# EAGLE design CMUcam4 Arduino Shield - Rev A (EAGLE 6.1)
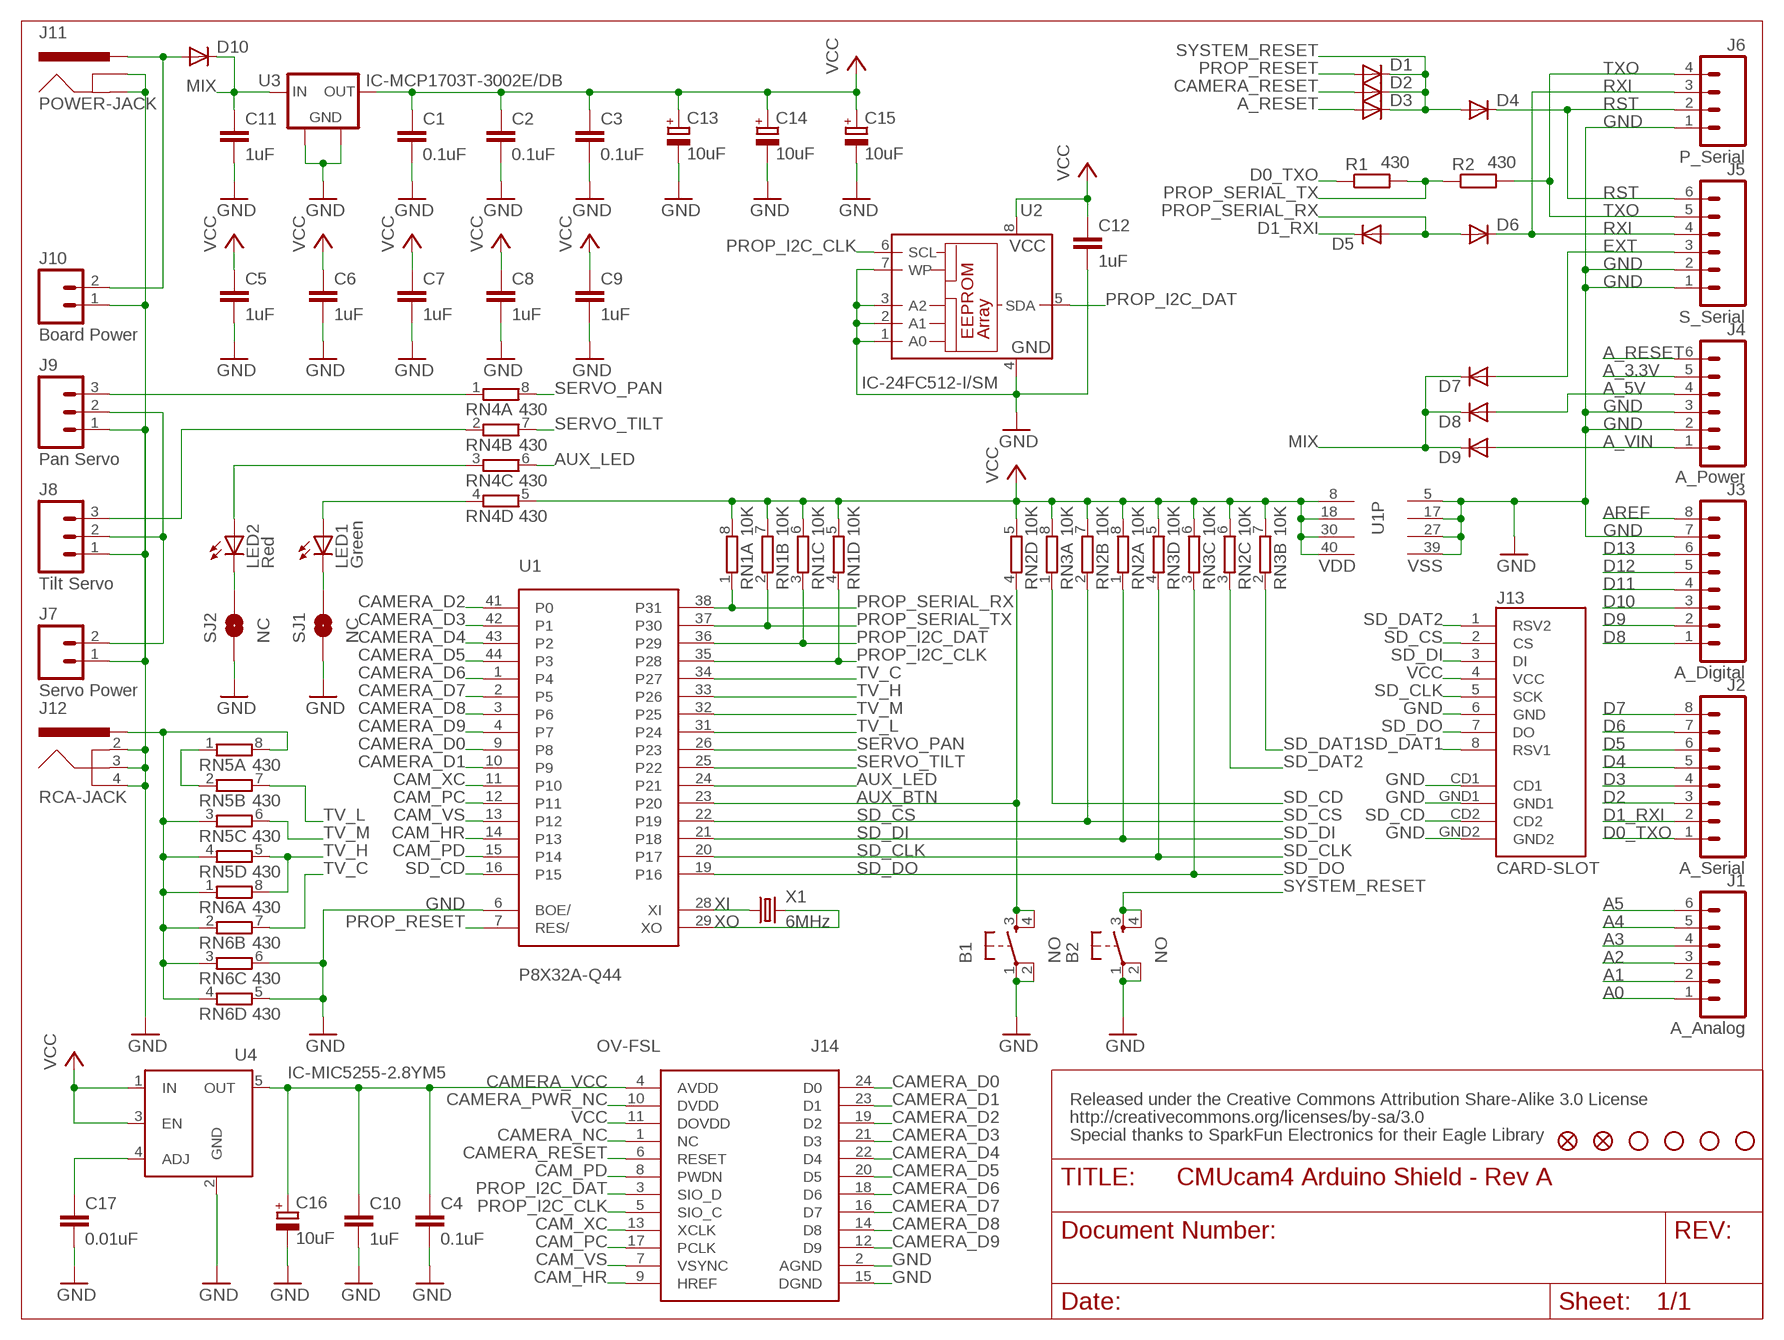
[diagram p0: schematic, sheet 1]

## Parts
B1  NO  PUSH-BUTTON  [PUSH-BUTTON]
B2  NO  PUSH-BUTTON  [PUSH-BUTTON]
C1  0.1uF  C-EUC0603K  [C0603K]
C2  0.1uF  C-EUC0603K  [C0603K]
C3  0.1uF  C-EUC0603K  [C0603K]
C4  0.1uF  C-EUC0603K  [C0603K]
C5  1uF  C-EUC0603K  [C0603K]
C6  1uF  C-EUC0603K  [C0603K]
C7  1uF  C-EUC0603K  [C0603K]
C8  1uF  C-EUC0603K  [C0603K]
C9  1uF  C-EUC0603K  [C0603K]
C10  1uF  C-EUC0603K  [C0603K]
C11  1uF  C-EUC0603K  [C0603K]
C12  1uF  C-EUC0603K  [C0603K]
C13  10uF  CPOL-EUA/3216-18R  [A/3216-18R]
C14  10uF  CPOL-EUA/3216-18R  [A/3216-18R]
C15  10uF  CPOL-EUA/3216-18R  [A/3216-18R]
C16  10uF  CPOL-EUA/3216-18R  [A/3216-18R]
C17  0.01uF  C-EUC0603K  [C0603K]
D1  DIODE-SOD523  [SOD523]
D2  DIODE-SOD523  [SOD523]
D3  DIODE-SOD523  [SOD523]
D4  DIODE-SOD523  [SOD523]
D5  DIODE-SOD523  [SOD523]
D6  DIODE-SOD523  [SOD523]
D7  DIODE-SOD323-R  [SOD323]
D8  DIODE-SOD323-R  [SOD323]
D9  DIODE-SOD323-R  [SOD323]
D10  DIODE-SOD323-R  [SOD323]
FID1  FIDUCIAL1X2  [FIDUCIAL-1X2]
FID2  FIDUCIAL1X2  [FIDUCIAL-1X2]
J1  A_Analog  M06SIP  [1X06]
J2  A_Serial  M081X08  [1X08]
J3  A_Digital  M081X08  [1X08]
J4  A_Power  M06SIP  [1X06]
J5  S_Serial  M06SIP  [1X06]
J6  P_Serial  M04PTH  [1X04]
J7  Servo Power  M02PTH  [1X02]
J8  Tilt Servo  M03PTH  [1X03]
J9  Pan Servo  M03PTH  [1X03]
J10  Board Power  M02PTH  [1X02]
J11  POWER-JACK  [POWER-JACK]
J12  RCA-JACK  [RCA-JACK]
J13  CARD-SLOT  [CARD-SLOT]
J14  OV-FSL  [OV-FSL]
LED1  Green  LEDCHIP-LED0603  [CHIP-LED0603]
LED2  Red  LEDCHIP-LED0603  [CHIP-LED0603]
R1  430  R-EU_R0603  [R0603]
R2  430  R-EU_R0603  [R0603]
RN1  10K  4R-N0603-ARV  [0603-ARV]
RN2  10K  4R-N0603-ARV  [0603-ARV]
RN3  10K  4R-N0603-ARV  [0603-ARV]
RN4  430  4R-N0603-ARV  [0603-ARV]
RN5  430  4R-N0603-ARV  [0603-ARV]
RN6  430  4R-N0603-ARV  [0603-ARV]
SJ1  NC  SOLDERJUMPERTRACE  [SJ_2S-TRACE]
SJ2  NC  SOLDERJUMPERTRACE  [SJ_2S-TRACE]
STD1  STAND-OFF  [STAND-OFF]
STD2  STAND-OFF  [STAND-OFF]
STD3  STAND-OFF  [STAND-OFF]
STD4  STAND-OFF  [STAND-OFF]
U1  P8X32A-Q44  [P8X32A-Q44]
U2  IC-24FC512-I/SM  [IC-SO-08M]
U3  IC-MCP1703T-3002E/DB  [IC-SOT-223]
U4  IC-MIC5255-2.8YM5  [IC-SOT-23-5]
X1  6MHz  CRYSTALHC49UP  [HC49UP]

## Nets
A0: J1.1
A1: J1.2
A2: J1.3
A3: J1.4
A4: J1.5
A5: J1.6
A_3.3V: J4.5
A_5V [vcc]: D8.A J4.4
A_RESET: D3.A J4.6
A_VIN: D9.A J4.1
AREF: J3.8
AUX_BTN: B1.3 B1.4 RN2.4 U1.23(P20)
AUX_LED: RN4.6 U1.24(P21)
BYP: C17.1 U4.4(ADJ)
CAM_HR: J14.9(HREF) U1.14(P13)
CAM_PC: J14.17(PCLK) U1.12(P11)
CAM_PD: J14.8(PWDN) U1.15(P14)
CAM_VS: J14.7(VSYNC) U1.13(P12)
CAM_XC: J14.13(XCLK) U1.11(P10)
CAMERA_D0: J14.24(D0) U1.9(P8)
CAMERA_D1: J14.23(D1) U1.10(P9)
CAMERA_D2: J14.19(D2) U1.41(P0)
CAMERA_D3: J14.21(D3) U1.42(P1)
CAMERA_D4: J14.22(D4) U1.43(P2)
CAMERA_D5: J14.20(D5) U1.44(P3)
CAMERA_D6: J14.18(D6) U1.1(P4)
CAMERA_D7: J14.16(D7) U1.2(P5)
CAMERA_D8: J14.14(D8) U1.3(P6)
CAMERA_D9: J14.12(D9) U1.4(P7)
CAMERA_NC: J14.1(NC)
CAMERA_PWR_NC: J14.10(DVDD)
CAMERA_RESET: D2.A J14.6(RESET)
CAMERA_VCC: C4.1 C10.1 C16.+ J14.4(AVDD) U4.5(OUT)
D0_TXO: J2.1 R1.1
D1_RXI: D5.C J2.2
D2: J2.3
D3: J2.4
D4: J2.5
D5: J2.6
D6: J2.7
D7: J2.8
D8: J3.1
D9: J3.2
D10: J3.3
D11: J3.4
D12: J3.5
D13: J3.6
EXT: D7.A J5.3
GND [vcc]: B1.1 B1.2 B2.1 B2.2 C1.2 C2.2 C3.2 C4.2 C5.2 C6.2 C7.2 C8.2 C9.2 C10.2 C11.2 C12.2 C13.- C14.- C15.- C16.- C17.2 J3.7 J4.2 J4.3 J5.1 J5.2 J6.1 J7.1 J8.1 J9.1 J10.1 J11.GND J11.GNDBREAK J12.2 J12.3 J12.4 J13.6(GND) J13.CD1 J13.GND1 J13.GND2 J14.2(AGND) J14.15(DGND) RN6.5 RN6.6 SJ1.1 SJ2.1 U1.5(VSS) U1.6(BOE/) U1.17(VSS) U1.27(VSS) U1.39(VSS) U2.1(A0) U2.2(A1) U2.3(A2) U2.4(GND) U2.7(WP) U3.2(GND) U3.4(FGND) U4.2(GND)
GREEN_BRIDGE: LED1.C SJ1.2
GREEN_CTRL: LED1.A RN4.4
MIX: C11.1 D7.C D8.C D9.C D10.C U3.1(IN)
PROP_I2C_CLK: J14.5(SIO_C) RN1.4 U1.35(P28) U2.6(SCL)
PROP_I2C_DAT: J14.3(SIO_D) RN1.3 U1.36(P29) U2.5(SDA)
PROP_RESET: D1.A U1.7(RES/)
PROP_SERIAL_RX: D5.A D6.A RN1.1 U1.38(P31)
PROP_SERIAL_TX: R1.2 R2.1 RN1.2 U1.37(P30)
RED_BRIDGE: LED2.C SJ2.2
RED_CTRL: LED2.A RN4.3
RST: D4.C J5.6 J6.2
RXI: D6.C J5.4 J6.3
SD_CD: J13.CD2 RN3.1 U1.16(P15)
SD_CLK: J13.5(SCK) RN3.4 U1.20(P17)
SD_CS: J13.2(CS) RN2.2 U1.22(P19)
SD_DAT1: J13.8(RSV1) RN3.2
SD_DAT2: J13.1(RSV2) RN2.3
SD_DI: J13.3(DI) RN2.1 U1.21(P18)
SD_DO: J13.7(DO) RN3.3 U1.19(P16)
SERVO_PAN: RN4.8 U1.26(P23)
SERVO_PAN_IO: J9.3 RN4.1
SERVO_PWR: J7.2 J8.2 J9.2
SERVO_TILT: RN4.7 U1.25(P22)
SERVO_TILT_IO: J8.3 RN4.2
SYSTEM_RESET: B2.3 B2.4 D1.C D2.C D3.C D4.A
SYSTEM_VIN: D10.A J10.2 J11.PWR
TV: J12.1 RN5.3 RN5.4 RN5.8 RN6.1 RN6.2 RN6.3 RN6.4
TV_C: RN6.7 U1.34(P27)
TV_H: RN5.5 RN6.8 U1.33(P26)
TV_L: RN5.7 U1.31(P24)
TV_M: RN5.6 U1.32(P25)
TV_R: RN5.1 RN5.2
TXO: J5.5 J6.4 R2.2
VCC: C1.1 C2.1 C3.1 C5.1 C6.1 C7.1 C8.1 C9.1 C12.1 C13.+ C14.+ C15.+ J13.4(VCC) J14.11(DOVDD) RN1.5 RN1.6 RN1.7 RN1.8 RN2.5 RN2.6 RN2.7 RN2.8 RN3.5 RN3.6 RN3.7 RN3.8 RN4.5 U1.8(VDD) U1.18(VDD) U1.30(VDD) U1.40(VDD) U2.8(VCC) U3.3(OUT) U4.1(IN) U4.3(EN)
XI: U1.28(XI) X1.1
XO: U1.29(XO) X1.2

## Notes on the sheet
- Released under the Creative Commons Attribution Share-Alike 3.0 License
- http://creativecommons.org/licenses/by-sa/3.0
- Special thanks to SparkFun Electronics for their Eagle Library

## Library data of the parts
B1 B2 = custom-jacks:PUSH-BUTTON
C1-C12 C17 = resistor:C-EU: CAPACITOR, European symbol
C13-C16 = resistor:CPOL-EU: POLARIZED CAPACITOR, European symbol
D1-D10 = diode:DIODE-: DIODE
FID1 FID2 = SparkFun:FIDUCIAL: Fiducial Alignment Points
J1 J4 J5 = SparkFun:M06: Header 6 Standard 6-pin 0.1" header. Use with straight break away headers (SKU : PRT-00116), right angle break away headers (PRT-00553), swiss pins (PRT-00743), machine pins (PRT-00117), and female headers (PRT-00115). Molex polarized connector foot print use with SKU : PRT-08094 with associated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
J2 J3 = SparkFun:M08: Header 8 Standard 8-pin 0.1" header. Use with straight break away headers (SKU : PRT-00116), right angle break away headers (PRT-00553), swiss pins (PRT-00743), machine pins (PRT-00117), and female headers (PRT-00115).
J6 = SparkFun:M04: Header 4 Standard 4-pin 0.1" header. Use with straight break away headers (SKU : PRT-00116), right angle break away headers (PRT-00553), swiss pins (PRT-00743), machine pins (PRT-00117), and female headers (PRT-00115). Molex polarized connector foot print use with SKU : PRT-08231 with associated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
J7 J10 = SparkFun:M02: Header 2
J8 J9 = SparkFun:M03: Header 3 Standard 3-pin 0.1" header. Use with straight break away headers (SKU : PRT-00116), right angle break away headers (PRT-00553), swiss pins (PRT-00743), machine pins (PRT-00117), and female headers (PRT-00115). Molex polarized connector foot print use with SKU : PRT-08232 with associated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
J11 = custom-jacks:POWER-JACK
J12 = custom-jacks:RCA-JACK
J13 = custom-jacks:CARD-SLOT
J14 = ovt-breakout:OV-FSL
LED1 LED2 = led:LED: LED
R1 R2 = resistor:R-EU_: RESISTOR, European symbol
RN1-RN6 = resistor-dil:4R-N: Array Chip Resistor Source: RS Component / Phycomp; OC_FARNELL: unknown; OC_NEWARK: unknown
SJ1 SJ2 = SparkFun:SOLDERJUMPER: Solder Jumper
STD1-STD4 = SparkFun:STAND-OFF: Stand Off
U1 = parallax-propeller:P8X32A-Q44
U2 = custom-jacks:IC-24FC512-I/SM
U3 = custom-jacks:IC-MCP1703T-3002E/DB
U4 = custom-jacks:IC-MIC5255-2.8YM5
X1 = crystal:CRYSTAL: CRYSTAL; OC_FARNELL: unknown; OC_NEWARK: unknown

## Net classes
0 default: width 0.203 mm
1 vcc: width 0.254 mm

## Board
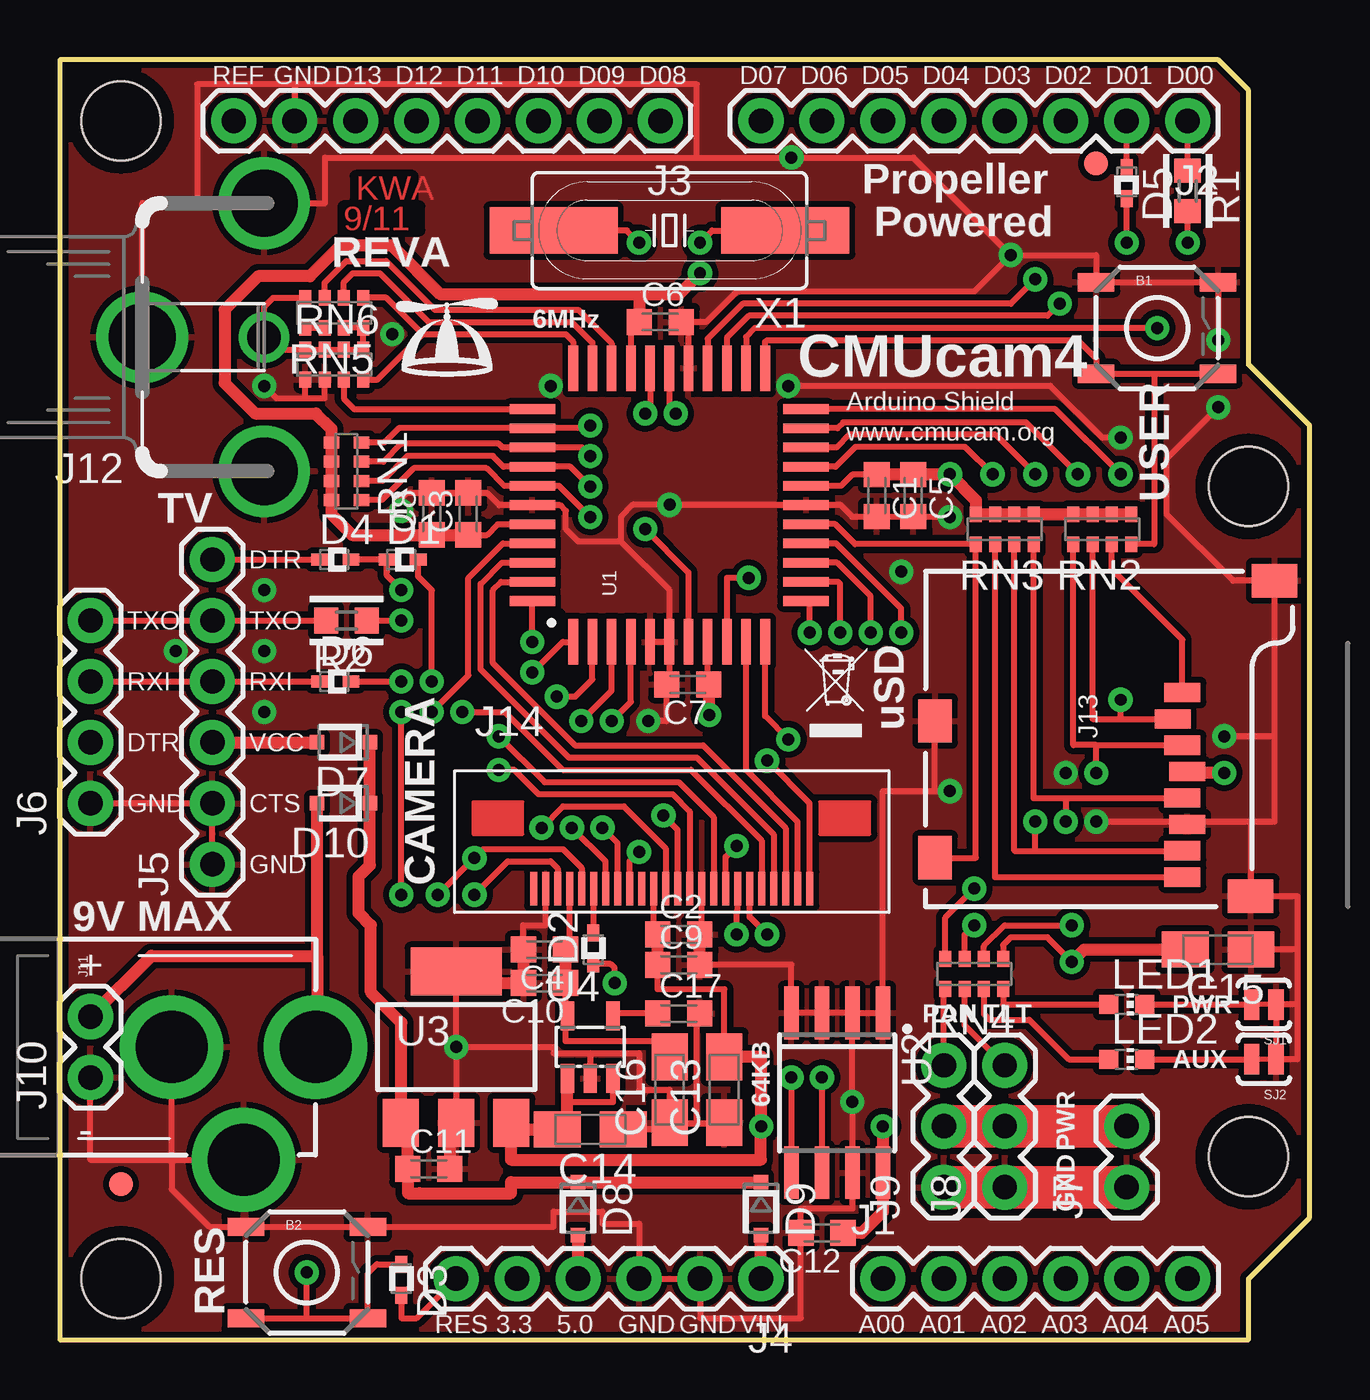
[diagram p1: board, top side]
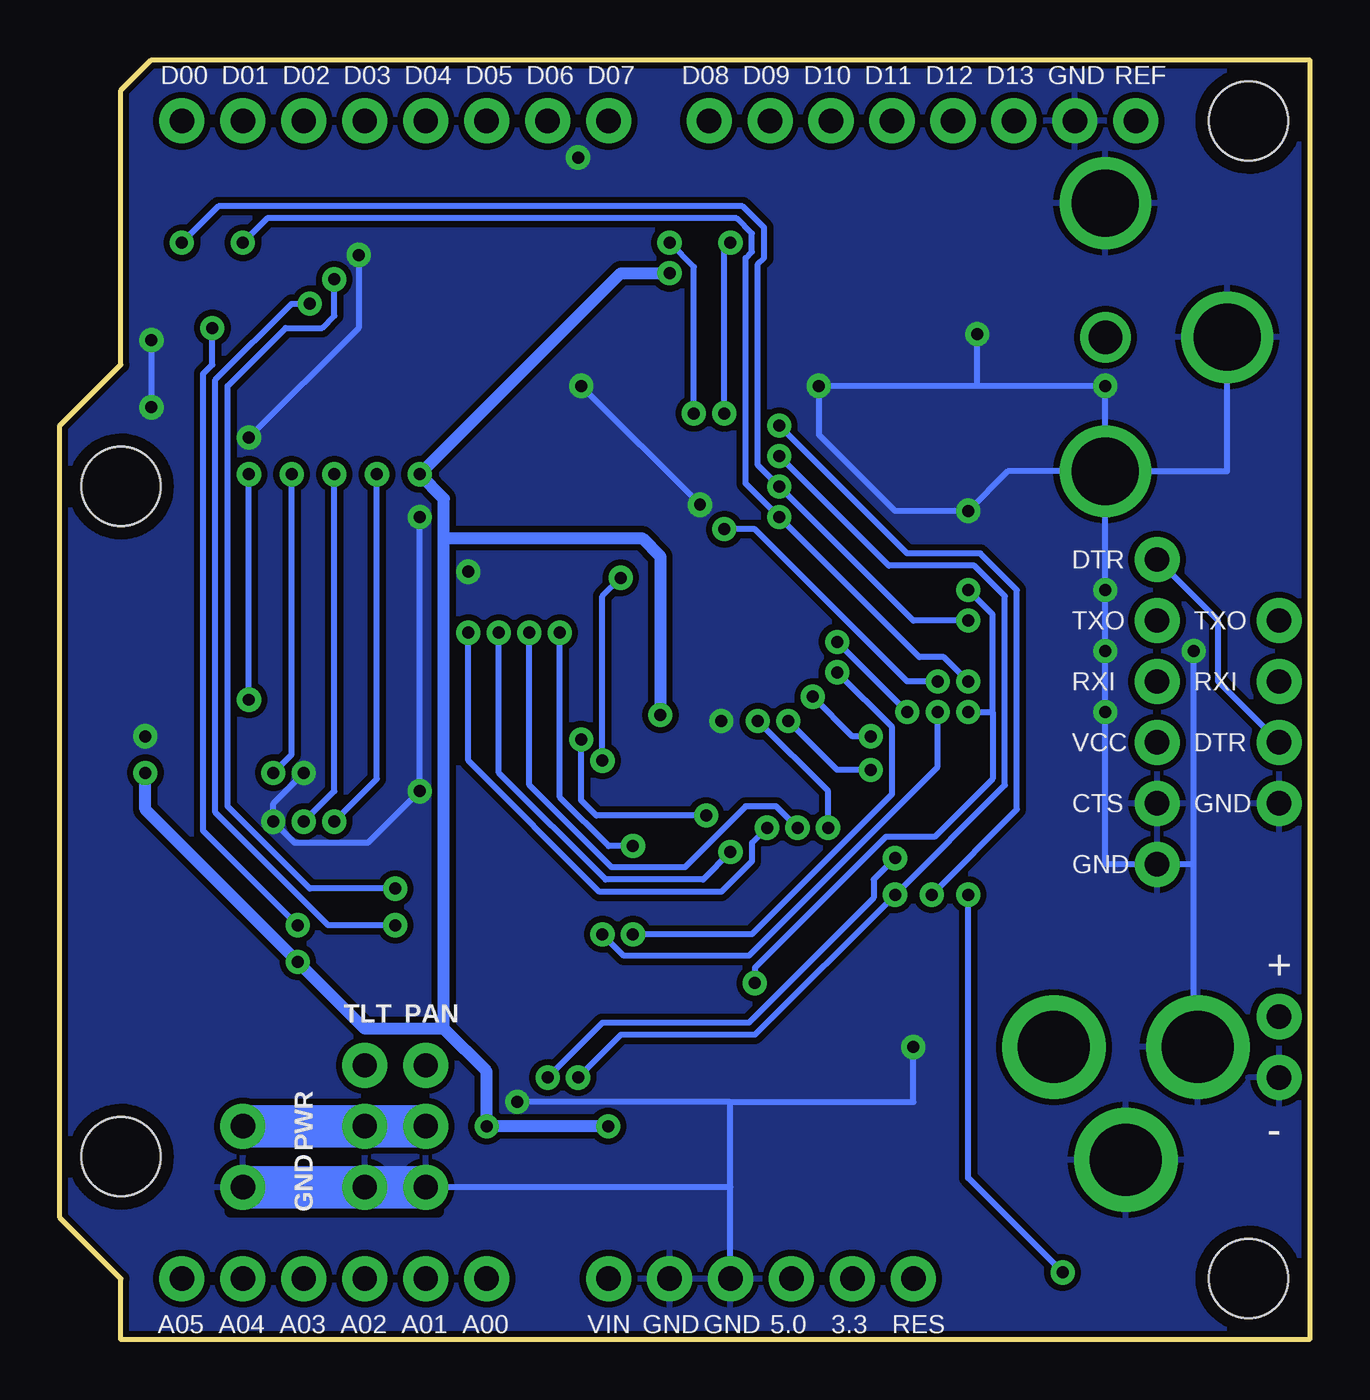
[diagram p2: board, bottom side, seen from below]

Size 52.07 x 53.34 mm. Coordinates in mm from the lower left corner, seen from the top.
Outline: 0,53.34 0,0 49.53,0 49.53,2.54 52.07,5.08 52.07,38.1 49.53,40.64 49.53,52.07 48.26,53.34 0,53.34
Copper layers (1*16): Top 0.035mm / dielectric 1.5mm / Bottom 0.035mm
Design rules: minimum track width 8mil, minimum drill 20mil, track to track 8mil, track to pad 8mil, pad to pad 8mil, via to via 8mil, smd to smd 8mil, copper to edge 10mil, drill to drill 8mil, minimum pad ring 12mil, minimum via ring 10mil, stop-mask expansion 4mil, vias tented up to drill 25mil, thermal gap 10mil
tRestrict: area 2,11.9 to 2.3,12.4; area 40.4,7.4 to 43.4,7.6; area 36.3,5.3 to 44.7,5.6; area 44.7,5.3 to 45,5.6; area 15.2,8.1 to 15.5,9.9; area 26.3,17.7 to 26.5,17.9; area 20.6,17 to 20.8,17.8; area 33.5,5.3 to 33.8,5.6; area 24.9,27.9 to 25.1,28.2; area 25.7,29.7 to 25.9,30; area 20.6,30 to 20.8,30.2; area 10.5,38.9 to 10.8,39.1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
bRestrict: area 2,11.9 to 2.3,12.4; area 40.4,7.4 to 43.4,7.6; area 36.3,5.3 to 44.7,5.6; area 44.7,5.3 to 45,5.6

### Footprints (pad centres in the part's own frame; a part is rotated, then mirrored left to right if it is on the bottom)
PUSH-BUTTON = smd 1.524 x 0.762: 1 -2.54,1.905; 2 2.54,1.905; 3 -2.54,-1.905; 4 2.54,-1.905
C0603K = smd 1.05 x 1.08: 1 -0.875,0; 2 0.875,0
A/3216-18R = smd 1.95 x 1.5: + 1.375,0; - -1.375,0
SOD523 = smd 0.7 x 0.5: A 0.7,0; C -0.6,0
SOD323 = smd 0.6 x 0.6: A 1.1,0; C -1.1,0
FIDUCIAL-1X2 = smd 1 x 1: 1 0,0
1X06 = drill 1.016 pad 1.88: 1 0,0; 2 2.54,0; 3 5.08,0; 4 7.62,0; 5 10.16,0; 6 12.7,0
1X08 = drill 1.016 pad 1.88: 1 0,0; 2 2.54,0; 3 5.08,0; 4 7.62,0; 5 10.16,0; 6 12.7,0; 7 15.24,0; 8 17.78,0
1X04 = drill 1.016 pad 1.88: 1 0,0; 2 2.54,0; 3 5.08,0; 4 7.62,0
1X02 = drill 1.016 pad 1.88: 1 0,0; 2 2.54,0
1X03 = drill 1.016 pad 1.88: 1 0,0; 2 2.54,0; 3 5.08,0
POWER-JACK = drill 2.997 pad 4.318: GND 0,7.7; GNDBREAK 4.7,10.7; PWR 0,13.7
RCA-JACK = drill 1.4: 1 0,0 | drill 2.8: 2 -5.588,0; 3 0,5.08; 4 5.588,0
CARD-SLOT = smd 0.8 x 1.5: 1 -8.94,10.7; 2 -7.84,10.3; 3 -6.74,10.7; 4 -5.64,10.9; 5 -4.54,10.7; 6 -3.44,10.9; 7 -2.34,10.7; 8 -1.24,10.7 | smd 1.8 x 1.4: CD1 -7.75,0.4; CD2 -2.05,0.4 | smd 1.4 x 1.9: GND1 -13.6,14.55; GND2 -0.45,13.55
OV-FSL = smd 0.3 x 1.4: 1 -5.15,-2.54; 2 -4.65,-2.54; 3 -4.15,-2.54; 4 -3.65,-2.54; 5 -3.15,-2.54; 6 -2.65,-2.54; 7 -2.15,-2.54; 8 -1.65,-2.54; 9 -1.15,-2.54; 10 -0.65,-2.54; 11 -0.15,-2.54; 12 0.35,-2.54; 13 0.85,-2.54; 14 1.35,-2.54; 15 1.85,-2.54; 16 2.35,-2.54; 17 2.85,-2.54; 18 3.35,-2.54; 19 3.85,-2.54; 20 4.35,-2.54; 21 4.85,-2.54; 22 5.35,-2.54; 23 5.85,-2.54; 24 6.35,-2.54
CHIP-LED0603 = smd 0.8 x 0.8: A 0,-0.75; C 0,0.75
R0603 = smd 1 x 1.1: 1 -0.85,0; 2 0.85,0
0603-ARV = smd 0.5 x 0.65: 1 -1.2,-0.625; 2 -0.4,-0.625; 3 0.4,-0.625; 4 1.2,-0.625; 5 1.2,0.625; 6 0.4,0.625; 7 -0.4,0.625; 8 -1.2,0.625
SJ_2S-TRACE = smd 0.635 x 1.27: 1 -0.508,0; 2 0.508,0
STAND-OFF = hole 3.302: 0,0
P8X32A-Q44 = smd 1.9 x 0.4: 1 -5.713,4.013; 2 -5.713,3.212; 3 -5.713,2.413; 4 -5.713,1.613; 5 -5.713,0.812; 6 -5.713,0.013; 7 -5.713,-0.787; 8 -5.713,-1.587; 9 -5.713,-2.388; 10 -5.713,-3.188; 11 -5.713,-3.987; 23 5.688,-3.987; 24 5.688,-3.188; 25 5.688,-2.388; 26 5.688,-1.587; 27 5.688,-0.787; 28 5.688,0.013; 29 5.688,0.812; 30 5.688,1.613; 31 5.688,2.413; 32 5.688,3.212; 33 5.688,4.013 | smd 0.4 x 1.9: 12 -4.013,-5.688; 13 -3.212,-5.688; 14 -2.413,-5.688; 15 -1.613,-5.688; 16 -0.812,-5.688; 17 -0.013,-5.688; 18 0.787,-5.688; 19 1.587,-5.688; 20 2.388,-5.688; 21 3.188,-5.688; 22 3.987,-5.688; 34 3.987,5.713; 35 3.188,5.713; 36 2.388,5.713; 37 1.587,5.713; 38 0.787,5.713; 39 -0.013,5.713; 40 -0.812,5.713; 41 -1.613,5.713; 42 -2.413,5.713; 43 -3.212,5.713; 44 -4.013,5.713
IC-SO-08M = smd 0.6 x 2.2: 1 -1.905,-3.33; 2 -0.635,-3.33; 3 0.635,-3.33; 4 1.905,-3.33; 5 1.905,3.33; 6 0.635,3.33; 7 -0.635,3.33; 8 -1.905,3.33
IC-SOT-223 = smd 1.5 x 2: 1 -2.3,-3.15; 2 0,-3.15; 3 2.3,-3.15 | smd 3.8 x 2: 4 0,3.15
IC-SOT-23-5 = smd 0.55 x 1.2: 1 -0.95,-1.3; 2 0,-1.3; 3 0.95,-1.3; 4 0.95,1.3; 5 -0.95,1.3
HC49UP = smd 5.334 x 1.93: 1 -4.826,0; 2 4.826,0

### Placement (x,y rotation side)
B1  45.72,42.16 0 top
B2  10.29,2.79 0 top
C1  34.04,35.18 270 top
C2  25.78,16.89 0 top
C3  17.02,34.42 90 top
C4  20.19,16.26 180 top
C5  35.56,35.18 270 top
C6  25.02,42.42 0 top
C7  26.16,27.3 180 top
C8  15.49,34.42 90 top
C9  25.78,15.62 0 top
C10  20.19,14.86 180 top
C11  15.37,7.11 0 top
C12  31.75,4.45 180 top
C13  27.69,10.41 90 top
C14  22.1,8.76 180 top
C15  48.26,16.26 180 top
C16  25.4,10.41 90 top
C17  25.78,13.59 0 top
D1  14.22,32.51 0 top
D2  22.23,16.26 90 top
D3  14.22,2.54 270 top
D4  11.43,32.51 0 top
D5  44.45,48.26 270 top
D6  11.43,27.43 0 top
D7  11.81,24.89 180 top
D8  21.59,5.46 270 top
D9  29.21,5.46 270 top
D10  11.81,22.35 180 top
FID1  43.18,49.02 0 top
FID2  2.54,6.48 0 top
J1  34.29,2.54 0 top
J2  46.99,50.8 180 top
J3  25.02,50.8 180 top
J4  29.21,2.54 180 top
J5  6.35,19.81 90 top
J6  1.27,22.35 90 top
J7  44.45,6.35 90 top
J8  39.37,6.35 90 top
J9  36.83,6.35 90 top
J10  1.27,10.92 90 top
J11  -3.05,12.19 270 top
J12  8.51,41.78 90 top
J13  36.07,18.03 270 top
J14  24.89,21.34 0 top
LED1  44.45,13.97 270 top
LED2  44.45,11.68 270 top
R1  46.99,47.88 270 top
R2  11.94,29.97 180 top
RN1  11.94,36.2 90 top
RN2  43.43,33.78 0 top
RN3  39.37,33.78 0 top
RN4  38.1,15.24 0 top
RN5  11.43,42.8 0 top
RN6  11.43,40.64 180 top
SJ1  50.16,13.97 180 top
SJ2  50.16,11.68 180 top
STD1  2.54,50.8 0 top
STD2  49.53,7.62 0 top
STD3  49.53,35.56 0 top
STD4  2.54,2.54 0 top
U1  25.4,34.8 90 top
U2  32.38,10.29 180 top
U3  16.51,12.19 0 top
U4  22.1,12.19 0 top
X1  25.4,46.23 180 top

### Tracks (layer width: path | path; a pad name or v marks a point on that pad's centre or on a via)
A_5V
  Top 0.508: J4.4 D8.A
A_RESET
  Top 0.254: D3.A 14.22,0.89 14.86,0.89 J4.6
A_VIN
  Top 0.508: J4.1 D9.A
AUX_BTN
  Top 0.254: 45.59,40.26 B1.3 43.18,40.89 42.42,41.66 29.46,41.66 29.39,41.58 U1.23 | 45.59,40.26 B1.4 | RN2.4 45.59,33.16 45.59,40.26
AUX_LED  (via drill 0.5)
  Top 0.254: U1.24 28.59,41.8 28.96,42.16 v45.72,42.16 | v42.16,17.27 39.37,17.27 38.5,16.4 RN4.6
  Bottom 0.254: v45.72,42.16 45.72,40.64 46.1,40.26 46.1,21.21 v42.16,17.27
BYP
  Top 0.254: C17.1 23.05,13.59 U4.4
CAM_HR  (via drill 0.5)
  Top 0.254: J14.9 23.74,19.93 v24.13,20.32 | v33.78,29.46 33.78,30.99 32.38,32.39 U1.14
  Bottom 0.254: v24.13,20.32 25.27,19.18 29.34,19.18 33.78,23.62 v33.78,29.46
CAM_PC  (via drill 0.5)
  Top 0.254: v31.24,29.46 31.24,30.79 U1.12 | v28.19,20.57 27.74,20.12 J14.17
  Bottom 0.254: v31.24,29.46 31.24,22.61 29.21,20.57 v28.19,20.57
CAM_PD  (via drill 0.5)
  Top 0.254: U1.15 32.35,33.19 35.05,30.48 v35.05,29.46 | J14.8 23.24,20.7 v22.61,21.34
  Bottom 0.254: v35.05,29.46 35.05,24.13 29.59,18.67 24.51,18.67 23.24,19.94 23.24,20.7 v22.61,21.34
CAM_VS  (via drill 0.5)
  Top 0.254: J14.7 22.74,19.93 v21.34,21.34 | U1.13 32.42,31.59 32.51,31.5 v32.51,29.46
  Bottom 0.254: v32.51,29.46 32.51,23.11 29.08,19.68 26.04,19.68 23.5,22.23 22.23,22.23 v21.34,21.34
CAM_XC  (via drill 0.5)
  Top 0.254: J14.13 25.74,21.25 v25.15,21.84 | U1.11 29.39,25.98 v30.35,25.02
  Bottom 0.254: v30.35,25.02 30.35,22.48 29.72,21.84 v25.15,21.84
CAMERA_D0  (via drill 0.5)
  Top 0.254: J14.24 31.24,22.35 v29.46,24.13 | v28.7,31.75 27.79,31.75 U1.9
  Bottom 0.254: v29.46,24.13 29.46,30.99 v28.7,31.75
CAMERA_D1
  Top 0.254: J14.23 30.74,21.58 28.59,23.74 U1.10
CAMERA_D2  (via drill 0.5)
  Top 0.254: U1.41 18.45,33.19 17.02,31.75 17.02,27.69 v15.49,26.16 | J14.19 28.74,17.61 v29.46,16.89
  Bottom 0.254: v15.49,26.16 15.49,23.88 23.37,16 28.57,16 v29.46,16.89
CAMERA_D3
  Top 0.254: J14.21 29.74,21.06 26.54,24.26 21.21,24.26 17.53,27.94 17.53,31.5 18.42,32.39 U1.42
CAMERA_D4
  Top 0.254: J14.22 30.24,21.32 26.8,24.77 21.46,24.77 18.03,28.19 18.03,31.24 18.38,31.59 U1.43
CAMERA_D5  (via drill 0.5)
  Top 0.254: v16.76,26.16 18.54,26.16 20.95,23.75 26.29,23.75 29.24,20.8 J14.20 | 19.81,30.79 U1.44 v19.68,29.08
  Bottom 0.254: v16.76,26.16 v19.68,29.08
CAMERA_D6  (via drill 0.5)
  Top 0.254: J14.18 28.24,17.83 28.19,17.83 v28.19,16.89 | U1.1 20.96,29.09 v19.68,27.81
  Bottom 0.254: v28.19,16.89 23.24,16.89 17.4,22.73 17.4,25.53 v19.68,27.81
CAMERA_D7  (via drill 0.5)
  Top 0.254: J14.16 27.24,21.78 25.78,23.24 20.19,23.24 v18.29,25.15 | U1.2 22.19,27.52 21.46,26.8 v20.7,26.8
  Bottom 0.254: v20.7,26.8 19.05,25.15 v18.29,25.15
CAMERA_D8  (via drill 0.5)
  Top 0.254: v18.29,23.75 18.92,23.75 19.94,22.73 25.53,22.73 26.24,22.02 J14.14 | U1.3 22.99,27.05 v21.72,25.78
  Bottom 0.254: v21.72,25.78 19.68,23.75 v18.29,23.75
CAMERA_D9  (via drill 0.5)
  Top 0.254: J14.12 25.24,20.48 23.5,22.23 20.95,22.23 v20.07,21.34 | U1.4 23.79,26.58 v22.99,25.78
  Bottom 0.254: v20.07,21.34 20.07,22.86 v22.99,25.78
CAMERA_RESET
  Top 0.254: J14.6 22.24,16.96 D2.A
CAMERA_VCC
  Top 0.254: J14.4 21.24,16.26 C4.1 | 21.07,13.49 C10.1 | C16.+ 25.4,12.45 21.07,12.45 21.07,13.49 | 21.07,13.49 U4.5
  Top 0.508: C10.1 C4.1
D0_TXO
  Top 0.254: R1.1 J2.1
D1_RXI
  Top 0.254: D5.C J2.2
EXT
  Top 0.508: J5.3 D7.A
GND  (via drill 0.5)
  Top 0.254: U1.6 25.39,27.41 C7.2 25.27,27.3 25.27,25.78 v24.51,25.78 | U1.27 26.19,42.42 C6.2 26.92,42.42 28.19,43.69 38.1,43.69 v39.62,45.21 | C8.2 17.79,35.29 18.3,34.78 U1.39 20.84,34.78 21.08,34.54 21.08,33.78 21.59,33.27 23.37,33.27 | 31.24,34.8 30.99,34.8 | 31.24,34.8 32.51,34.8 33.01,34.3 C1.2 C5.2 | 4.65,7.49 J11.GND | 4.65,7.49 J11.GNDBREAK | J10.1 1.27,7.49 4.65,7.49 | J5.1 J5.2 J6.1 | J12.3 3.43,47.37 J12.4 11.05,47.37 11.05,49.28 26.54,49.28 | C8.2 16.51,35.29 | v39.62,45.21 35.56,49.28 v30.48,49.28 26.54,49.28 | 10.23,39.24 RN6.5 | U1.6 U1.5 | v25.4,34.8 25.39,34.78 | v25.4,34.8 31.07,34.8 U1.17 31.24,34.78 31.24,34.8 | v39.62,45.21 43.18,45.21 B1.1 B1.2 v48.26,41.66 | RN6.6 11.03,39.24 10.23,39.24 | 10.23,39.24 9.02,39.24 v8.51,39.75 | 9.78,52.32 5.71,52.32 5.71,47.37 | U2.2 U2.3 U2.4 30.48,15.62 C9.2 | U2.2 U2.1 34.29,22.86 36.45,22.86 | 4.65,7.49 4.65,6.27 6.22,4.7 B2.1 B2.2 20.57,4.7 20.57,5.33 22.61,5.33 22.61,4.83 24.13,4.83 J4.3 J4.2 26.67,0.89 30.88,0.89 C12.2 30.88,5.46 33.02,5.46 U2.7 v33.02,9.91 U2.2 | 9.78,52.32 J3.7 | 9.78,52.32 26.54,52.32 26.54,49.28 | v44.2,37.59 43.43,37.59 41.27,39.75 v30.35,39.75 | SJ2.1 SJ1.1 51.56,13.97 | v43.18,21.59 46.97,21.59 | 46.97,21.59 J13.6 | J14.15 26.74,16.89 C2.2 | J14.2 20.24,17.27 19.3,17.27 19.3,16.26 C4.2 | v16.51,12.19 U3.2 | v16.51,12.19 U3.4 | 50.62,25.15 J13.GND1 48.88,31.63 46.1,34.42 46.1,36.7 v48.26,38.86 | 49.62,21.59 50.62,21.59 50.62,25.15 | 50.62,25.15 v48.51,25.15 | 49.62,21.59 J13.GND2 51.56,18.48 51.56,16.26 | 46.97,21.59 49.62,21.59 | 51.56,16.26 51.56,13.97 | 51.56,16.26 C15.- | 50.8,11.68 51.56,11.68 51.56,13.97 | 36.45,22.86 v37.08,22.86
  Top 0.254: v37.08,34.29 C5.2 | U1.6 25.39,31.25 23.37,33.27 | 23.37,33.27 23.37,34.29 23.88,34.8 v25.4,34.8 | C8.2 C3.2 | v14.22,34.54 14.22,35.05 14.48,35.31 15.49,35.31 | 36.45,22.86 36.45,25.78 J13.CD1 | 22.1,11.94 24.13,11.94 24.13,10.41 25.4,10.41 C16.- 25.4,9.02 | 22.1,11.94 U4.2 | 26.54,9.02 27.69,9.02 C13.- | C14.- 23.5,8.76 25.4,8.76 25.4,9.02 | 26.54,9.02 26.54,13.59 C17.2 | 25.4,9.02 26.54,9.02 | 22.1,11.94 20.57,11.94 20.57,12.19 v16.51,12.19
  Top 0.508: C9.2 C2.2 | C4.2 C10.2 16.51,14.86 U3.4 | U3.2 16.24,9.04 C11.2
  Top 1.778: J7.1 J8.1 J9.1
  Bottom 0.254: J12.2 v8.51,39.75 13.84,39.75 | J12.2 12.57,36.2 v14.22,34.54 17.27,34.54 20.45,37.72 v20.45,39.75 13.84,39.75 | v44.2,37.59 39.62,42.16 v39.62,45.21 | v48.26,41.66 v48.26,38.86 | v30.35,39.75 v25.4,34.8 | v37.08,34.29 v37.08,22.86 39.24,20.7 42.29,20.7 v43.18,21.59 43.18,22.35 v41.91,23.62 | J4.3 24.13,6.35 | 24.13,6.35 J9.1 | 4.83,19.81 v4.83,28.7 | 4.83,19.81 J5.1 8.51,19.81 v8.51,26.16 v8.51,28.7 v8.51,31.24 J12.2 | 24.13,9.91 16.51,9.91 v16.51,12.19 | 13.84,39.75 v13.84,41.91 | 4.83,19.81 4.83,12.19 J11.GND | 24.13,6.35 24.13,9.91 | 24.13,9.91 v33.02,9.91 | J12.3 3.43,36.2 J12.2
  Bottom 1.778: J7.1 J8.1 J9.1
  other vias: 35.05,32
  pour Top (isolate 0.254): 0,53.34 52.07,53.34 52.07,0 0,0
  pour Bottom (isolate 0.254): 0,53.34 52.07,53.34 52.07,0 0,0
GREEN_BRIDGE
  Top 0.254: LED1.C SJ1.2
GREEN_CTRL
  Top 0.254: LED1.A 39.3,13.97 RN4.4
MIX
  Top 0.508: D7.C D10.C 12.91,19.77 12.45,19.3 12.45,17.78 12.95,17.27 12.95,14.48 14.22,13.21 14.22,9.06 U3.1 14.49,9.04 C11.1 14.49,6.1 14.62,6.1 14.99,6.1 18.8,6.1 18.8,6.56 D8.C D9.C
PROP_I2C_CLK  (via drill 0.5)
  Top 0.254: J14.5 21.74,19.66 20.95,20.45 17.65,20.45 v17.27,20.07 v15.75,18.54 | RN1.4 13.52,37.4 14.11,37.99 U1.35 21.98,37.99 v22.1,38.1 | v31.75,10.92 U2.6
  Bottom 0.254: v17.27,20.07 18.16,19.18 18.16,18.41 23.37,13.21 29.46,13.21 v31.75,10.92 | v22.1,38.1 16.76,32.77 13.72,32.77 12.19,31.24 12.19,22.1 v15.75,18.54
PROP_I2C_DAT  (via drill 0.5)
  Top 0.254: J14.3 20.74,19.64 20.45,19.94 18.67,19.94 v17.27,18.54 | RN1.3 13.48,36.59 14.22,37.34 18.29,37.34 18.44,37.19 U1.36 21.74,37.19 v22.1,36.83 | v30.48,10.92 U2.5
  Bottom 0.254: v30.48,10.92 28.7,12.7 23.11,12.7 v17.27,18.54 12.7,23.11 12.7,30.99 13.97,32.26 17.53,32.26 v22.1,36.83
PROP_RESET  (via drill 0.5)
  Top 0.254: D1.A 14.92,31.81 15.49,31.24 v15.49,27.43 | U1.7 26.19,31.98 v24.38,33.78
  Bottom 0.254: v15.49,27.43 16.76,27.43 23.11,33.78 v24.38,33.78
PROP_SERIAL_RX  (via drill 0.5)
  Top 0.254: RN1.1 13.4,34.99 14.73,36.32 17.78,36.32 18.52,35.59 U1.38 20.8,35.59 v22.1,34.29 | v44.45,45.72 D5.A | D6.A v14.22,27.43
  Bottom 0.254: v44.45,45.72 43.43,46.74 23.88,46.74 23.24,46.1 23.24,45.34 23.5,45.09 23.5,35.69 v22.1,34.29 16.26,28.45 15.24,28.45 v14.22,27.43
PROP_SERIAL_TX  (via drill 0.5)
  Top 0.254: RN1.2 13.44,35.8 14.48,36.83 18.03,36.83 18.48,36.39 U1.37 21.27,36.39 v22.1,35.56 | v46.99,45.72 R1.2 | R2.1 v14.22,29.97
  Bottom 0.254: v46.99,45.72 45.47,47.24 23.62,47.24 22.73,46.35 22.73,45.09 22.99,44.83 22.99,36.45 v22.1,35.56 16.51,29.97 v14.22,29.97
RED_BRIDGE
  Top 0.254: LED2.C SJ2.2
RED_CTRL
  Top 0.254: RN4.3 38.5,13.57 38.73,13.34 40.39,13.34 42.04,11.68 LED2.A
RST
  Top 0.254: J5.6 D4.C
  Bottom 0.254: J5.6 3.81,29.97 3.81,27.43 J6.2
RXI
  Top 0.254: J6.3 J5.4 D6.C
SD_CD
  Top 0.254: J13.CD2 38.17,20.08 RN3.1 33.14,33.16 32.31,33.99 U1.16
SD_CLK  (via drill 0.5)
  Top 0.254: RN3.4 40.57,22.57 41.91,22.57 | U1.20 32.36,37.19 32.89,37.72 38.99,37.72 v40.64,36.07 | 41.91,22.57 v41.91,21.59 | 41.91,22.57 J13.5
  Bottom 0.254: v40.64,36.07 40.64,22.86 v41.91,21.59
SD_CS  (via drill 0.5)
  Top 0.254: RN2.2 43.03,25.87 44.2,25.87 | 44.2,25.87 J13.2 | U1.22 41.48,38.78 v44.2,36.07 | 44.2,25.87 v44.2,26.67
  Bottom 0.254: v44.2,26.67 v44.2,36.07
SD_DAT1
  Top 0.254: RN3.2 38.97,19.27 J13.8
SD_DAT2
  Top 0.254: J13.1 46.77,29.18 43.83,32.11 RN2.3
SD_DI  (via drill 0.5)
  Top 0.254: RN2.1 42.23,24.77 43.18,24.77 | U1.21 32.4,37.99 32.64,38.23 40.26,38.23 v42.42,36.07 | v43.18,23.62 43.18,24.77 | 43.18,24.77 J13.3
  Bottom 0.254: v42.42,36.07 42.42,24.38 v43.18,23.62
SD_DO  (via drill 0.5)
  Top 0.254: RN3.3 39.77,20.37 40.64,20.37 | U1.19 32.32,36.39 33.15,37.21 37.72,37.21 v38.86,36.07 | 40.64,20.37 v40.64,21.59 | 40.64,20.37 J13.7
  Bottom 0.254: v38.86,36.07 38.86,23.37 v40.64,21.59
SERVO_PAN  (via drill 0.5)
  Top 0.254: U1.26 26.99,41.72 28.45,43.18 39.62,43.18 v40.64,44.2 | RN4.8 36.9,17.6 v38.1,18.8
  Bottom 0.254: v40.64,44.2 40.64,42.67 41.15,42.16 42.67,42.16 45.09,39.75 45.09,22.23 41.66,18.8 v38.1,18.8
SERVO_PAN_IO
  Top 0.254: RN4.1 36.83,14.62 J9.3
SERVO_PWR
  Top 1.778: J9.2 J8.2 J7.2
  Bottom 1.778: J9.2 J8.2 J7.2
SERVO_TILT  (via drill 0.5)
  Top 0.254: U1.25 27.79,41.76 28.7,42.67 41.15,42.67 v41.66,43.18 | RN4.7 37.7,16.87 v38.1,17.27
  Bottom 0.254: v41.66,43.18 42.42,43.18 45.59,40.01 45.59,21.97 40.89,17.27 v38.1,17.27
SERVO_TILT_IO
  Top 0.254: RN4.2 37.7,13.1 J8.3
SYSTEM_RESET  (via drill 0.5)
  Top 0.254: v23.11,14.86 23.11,15.49 22.95,15.66 D2.C | D1.C D4.A | D1.C 13.62,32 | v14.22,31.24 13.62,31.84 D1.C | v14.22,18.54 v14.22,26.16 | B2.3 10.29,0.89 | 10.29,0.89 B2.4 12.83,2.76 13.21,3.14 D3.C | 10.29,0.89 v10.29,2.79
  Bottom 0.254: v23.11,14.86 23.11,15.49 17.65,20.95 15.62,20.95 13.21,23.37 13.21,26.16 | v14.22,31.24 13.21,30.23 13.21,26.16 | v14.22,26.16 13.21,26.16 | v14.22,18.54 14.22,6.73 v10.29,2.79
SYSTEM_VIN
  Top 0.508: J10.2 3.81,16 10.71,16 | 10.71,16 D10.A | 10.71,16 10.71,12.19 J11.PWR
TV
  Top 0.254: RN5.3 RN5.4 RN6.1 RN6.2 RN6.3 RN6.4 9.03,41.27 J12.1 8.51,43.05 8.88,43.42 RN5.8
TV_C
  Top 0.254: U1.34 12.27,38.78 11.83,39.22 RN6.7
TV_H
  Top 0.254: 21.39,40.02 U1.33 21.39,41.6 21.08,41.91 15.11,41.91 | RN5.5 13.6,43.42 15.11,41.91 | RN6.8 13.22,40.02 15.11,41.91
TV_L
  Top 0.254: U1.31 22.99,41.53 21.59,42.93 15.62,42.93 13.59,44.96 11.94,44.96 11.03,44.05 RN5.7
TV_M
  Top 0.254: RN5.6 11.83,44.09 12.19,44.45 13.34,44.45 15.37,42.42 21.34,42.42 22.19,41.57 U1.32
TV_R
  Top 0.254: RN5.1 RN5.2
TXO
  Top 0.254: J6.4 J5.5 R2.2
VCC  (via drill 0.5)
  Top 0.254: U1.30 23.79,42.42 C6.1 | C3.1 17.79,33.54 18.24,33.99 U1.40 | U1.18 32.54,35.59 33.01,36.05 C1.1 | U1.8 26.99,27.3 C7.1 | 24.74,16.89 J14.11 | RN4.5 39.3,16.44 39.62,16.76 41.15,16.76 v42.16,15.75 | C5.1 35.57,36.07 | U4.3 23.05,9.91 21.15,9.91 | C9.1 24.91,14.61 27.69,14.61 C13.+
  Top 0.508: J13.4 47.02,23.62 v48.51,23.62 | 24.13,43.56 C6.1 | 24.13,43.56 15.88,43.56 13.84,45.59 11.68,45.59 10.41,44.32 8.26,44.32 6.86,42.93 6.86,39.88 8.13,38.61 10.67,38.61 11.31,37.96 RN1.5 RN1.6 RN1.7 RN1.8 11.31,34.41 12.18,33.54 C8.1 | RN2.5 RN2.6 RN2.7 RN2.8 RN3.5 RN3.6 RN3.7 RN3.8 38.17,34.98 v37.08,36.07 37.07,36.05 C5.1 C1.1 | 24.13,43.56 25.78,43.56 v26.67,44.45 | v34.29,8.89 U2.8 34.29,5.33 33.4,4.45 C12.1 | C8.1 16.51,33.54 | 18.8,8.76 18.8,7.49 29.21,7.49 29.21,8.89 v29.23,8.89 29.23,11.79 C13.+ | v42.16,15.75 42.67,16.26 C15.+ | v27.05,26.04 C7.1 | 18.8,8.76 18.8,9.04 U3.3 | 24.74,16.89 C2.1 C9.1 | U4.1 21.15,9.91 21.15,8.76 C14.+ | 18.8,8.76 C14.+ | C8.1 C3.1 | C14.+ 21.02,8.76
  Bottom 0.508: 36.07,12.95 39.37,12.95 v42.16,15.75 48.51,22.1 v48.51,23.62 | v26.67,44.45 28.7,44.45 v37.08,36.07 36.07,35.05 36.07,33.4 | 36.07,12.95 34.29,11.18 v34.29,8.89 v29.23,8.89 | 36.07,12.95 36.07,33.4 | v27.05,26.04 27.05,32.64 27.81,33.4 36.07,33.4
XI  (via drill 0.5)
  Top 0.254: X1.1 27.18,46.23 v26.67,45.72 | U1.28 25.39,38.87 v25.65,38.61
  Bottom 0.254: v25.65,38.61 25.65,44.7 v26.67,45.72
XO  (via drill 0.5)
  Top 0.254: X1.2 23.62,46.23 v24.13,45.72 | U1.29 24.59,38.81 v24.38,38.61
  Bottom 0.254: v24.38,38.61 24.38,45.47 v24.13,45.72

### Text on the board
Top: KWA | 9/11
tPlace: REF | GND | D13 | D12 | D11 | D10 | D09 | D08 | D07 | D06 | D05 | D04 | D03 | D02 | D01 | D00 | Propeller | Powered | REVA | 6MHz | CMUcam4 | Arduino Shield | www.cmucam.org | USER | TV | DTR | TXO | TXO | RXI | RXI | DTR | VCC | uSD | GND | CTS | GND | CAMERA | 9V MAX | + | PWR | PAN | TLT | 64KB | AUX | - | PWR | RES | GND | RES | 3.3 | 5.0 | GND | GND | VIN | A00 | A01 | A02 | A03 | A04 | A05
bPlace: REF | GND | D13 | D12 | D11 | D10 | D09 | D08 | D07 | D06 | D05 | D04 | D03 | D02 | D01 | D00 | DTR | TXO | TXO | RXI | RXI | DTR | VCC | GND | CTS | GND | + | PAN | TLT | - | PWR | GND | RES | 3.3 | 5.0 | GND | GND | VIN | A00 | A01 | A02 | A03 | A04 | A05
tDocu: Released under the Creative Commons Attribution Share-Alike 3.0 License | http://creativecommons.org/licenses/by-sa/3.0 | Special thanks to SparkFun Electronics for their Eagle Library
